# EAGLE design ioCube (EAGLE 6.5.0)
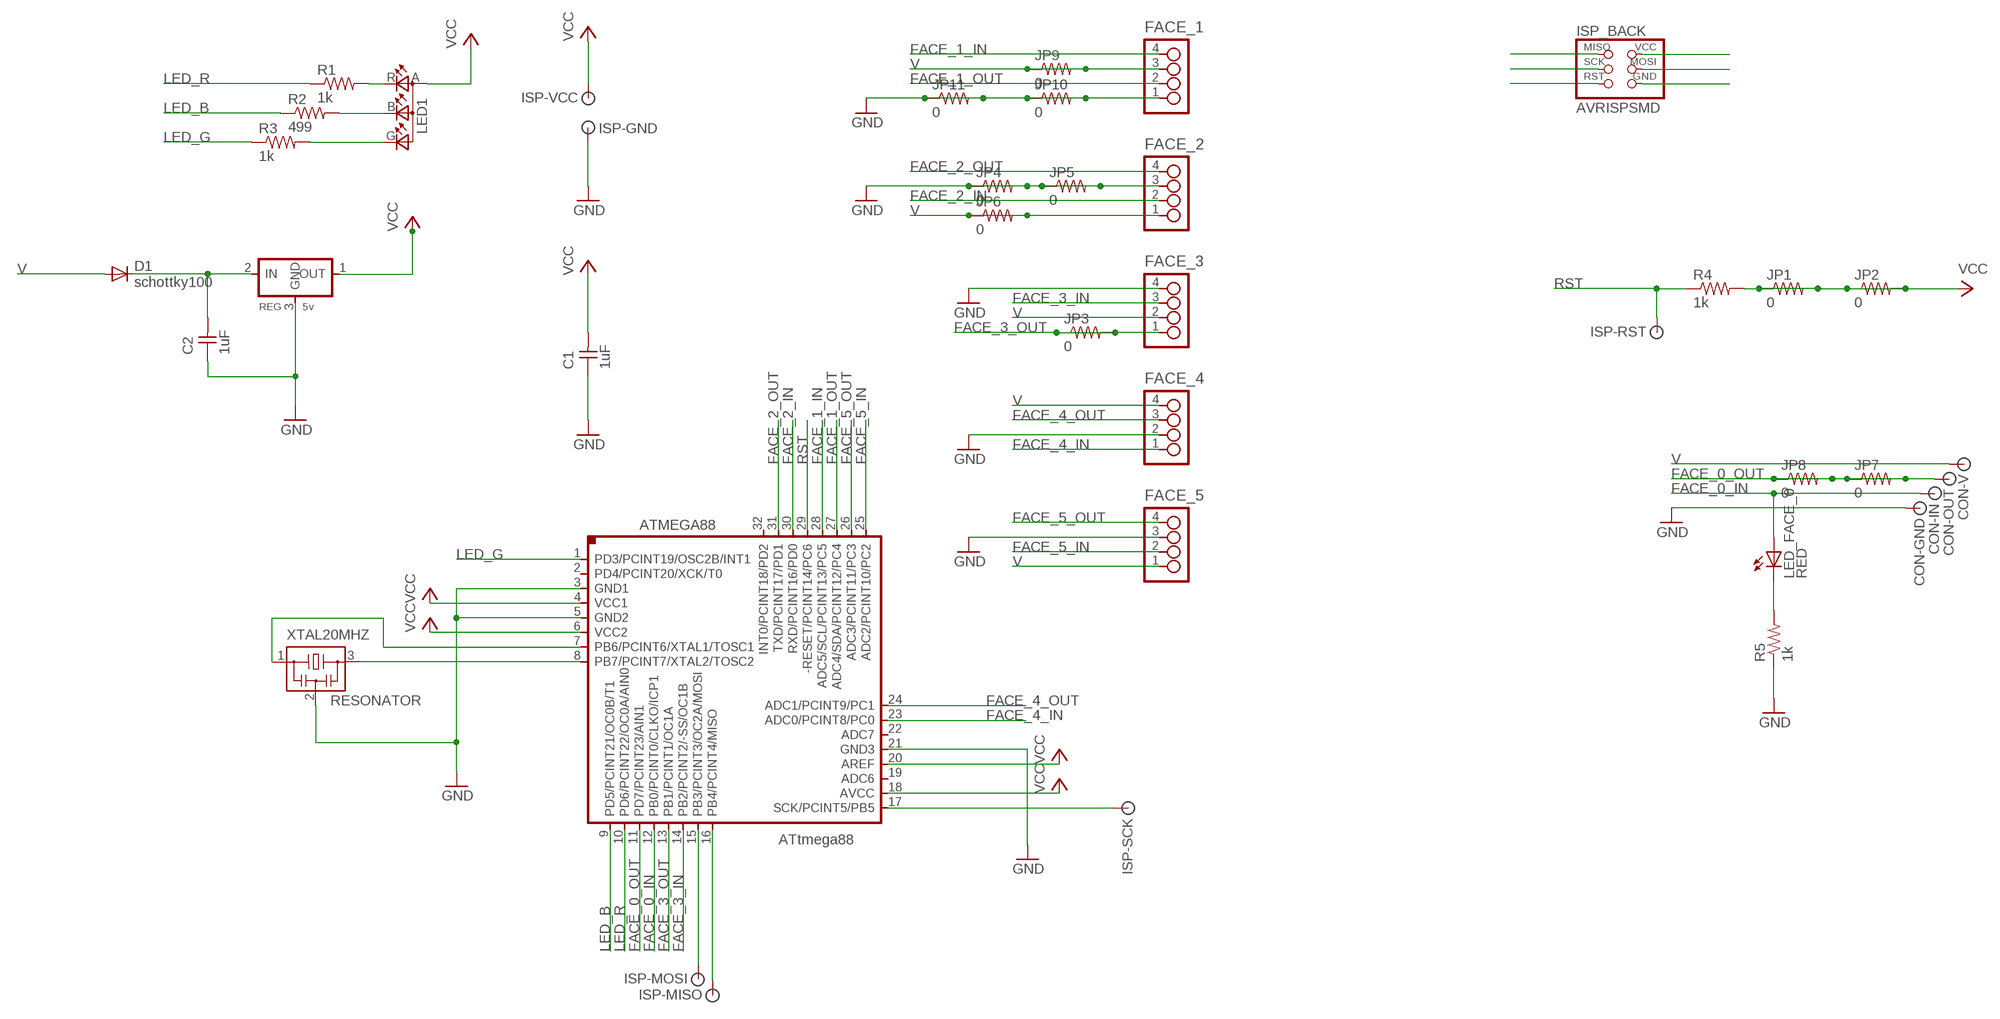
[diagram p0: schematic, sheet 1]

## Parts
ATMEGA88  ATMEGA88TQFP  [TQFP32-08]
C1  1uF  UNPOLARIZED_CAPACITOR1206  [1206]
C2  1uF  UNPOLARIZED_CAPACITOR1206  [1206]
CON-GND  SIGNAL  [PAD.2]
CON-IN  SIGNAL  [PAD.2]
CON-OUT  SIGNAL  [PAD.2]
CON-V  SIGNAL  [PAD.2]
D1  schottky100  DIODESOD123  [SOD123]
FACE_1  4_PIN_HEADER  [SMT_PINS_4]
FACE_2  4_PIN_HEADER  [SMT_PINS_4]
FACE_3  4_PIN_HEADER  [SMT_PINS_4]
FACE_4  4_PIN_HEADER  [SMT_PINS_4]
FACE_5  4_PIN_HEADER  [SMT_PINS_4]
ISP-GND  SIGNAL  [PAD.2]
ISP-MISO  SIGNAL  [PAD.2]
ISP-MOSI  SIGNAL  [PAD.2]
ISP-RST  SIGNAL  [PAD.2]
ISP-SCK  SIGNAL  [PAD.2]
ISP-VCC  SIGNAL  [PAD.2]
ISP_BACK  AVRISPSMD  [2X03SMD]
JP1  0  RESISTOR1206  [1206]
JP2  0  RESISTOR1206  [1206]
JP3  0  RESISTOR1206  [1206]
JP4  0  RESISTOR1206  [1206]
JP5  0  RESISTOR1206  [1206]
JP6  0  RESISTOR1206  [1206]
JP7  0  RESISTOR1206  [1206]
JP8  0  RESISTOR1206  [1206]
JP9  0  RESISTOR1206  [1206]
JP10  0  RESISTOR1206  [1206]
JP11  0  RESISTOR1206  [1206]
LED1  LEDRGBOLD  [P-LCC-4-3]
LED_FACE_0  RED  LED1206  [1206]
R1  1k  RESISTOR1206  [1206]
R2  499  RESISTOR1206  [1206]
R3  1k  RESISTOR1206  [1206]
R4  1k  RESISTOR1206  [1206]
R5  1k  RESISTOR1206  [1206]
REG  5v  REGULATORSOT23  [SOT23]
XTAL20MHZ  RESONATOR  [EFOBM]

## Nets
FACE_0_IN: ATMEGA88.12(PB0/PCINT0/CLKO/ICP1) CON-IN.P$1 LED_FACE_0.1(A)
FACE_0_OUT: ATMEGA88.11(PD7/PCINT23/AIN1) CON-OUT.P$1 JP7.1 JP7.2 JP8.1 JP8.2
FACE_1_IN: ATMEGA88.28(ADC5/SCL/PCINT13/PC5) FACE_1.4
FACE_1_OUT: ATMEGA88.27(ADC4/SDA/PCINT12/PC4) FACE_1.2
FACE_2_IN: ATMEGA88.30(RXD/PCINT16/PD0) FACE_2.2
FACE_2_OUT: ATMEGA88.31(TXD/PCINT17/PD1) FACE_2.4
FACE_3_IN: ATMEGA88.14(PB2/PCINT2/-SS/OC1B) FACE_3.3
FACE_3_OUT: ATMEGA88.13(PB1/PCINT1/OC1A) FACE_3.1 JP3.1 JP3.2
FACE_4_IN: ATMEGA88.23(ADC0/PCINT8/PC0) FACE_4.1
FACE_4_OUT: ATMEGA88.24(ADC1/PCINT9/PC1) FACE_4.3
FACE_5_IN: ATMEGA88.25(ADC2/PCINT10/PC2) FACE_5.2
FACE_5_OUT: ATMEGA88.26(ADC3/PCINT11/PC3) FACE_5.4
GND: ATMEGA88.3(GND1) ATMEGA88.5(GND2) ATMEGA88.21(GND3) C1.1 C2.1 CON-GND.P$1 FACE_1.1 FACE_2.3 FACE_3.4 FACE_4.2 FACE_5.3 ISP-GND.P$1 JP4.1 JP4.2 JP5.1 JP5.2 JP10.1 JP10.2 JP11.1 JP11.2 R5.1 REG.3(GND) XTAL20MHZ.2
LED_B: ATMEGA88.9(PD5/PCINT21/OC0B/T1) R2.1
LED_G: ATMEGA88.1(PD3/PCINT19/OSC2B/INT1) R3.1
LED_R: ATMEGA88.10(PD6/PCINT22/OC0A/AIN0) R1.1
N$1: ATMEGA88.8(PB7/PCINT7/XTAL2/TOSC2) XTAL20MHZ.3
N$2: ATMEGA88.7(PB6/PCINT6/XTAL1/TOSC1) XTAL20MHZ.1
N$3: ATMEGA88.17(SCK/PCINT5/PB5) ISP-SCK.P$1
N$4: ATMEGA88.16(PB4/PCINT4/MISO) ISP-MISO.P$1
N$5: ATMEGA88.15(PB3/PCINT3/OC2A/MOSI) ISP-MOSI.P$1
N$6: LED1.R(CRED) R1.2
N$7: LED_FACE_0.2(C) R5.2
N$8: LED1.B(CBLUE) R2.2
N$9: LED1.G(CGREEN) R3.2
N$10: ISP_BACK.2(VCC)
N$11: C2.2 D1.CATHODE(C) REG.2(IN)
N$12: ISP_BACK.4(MOSI)
N$13: ISP_BACK.6(GND)
N$14: ISP_BACK.1(MISO)
N$15: ISP_BACK.3(SCK)
N$16: ISP_BACK.5(RST)
RST: ATMEGA88.29(-RESET/PCINT14/PC6) ISP-RST.P$1 R4.1
V: CON-V.P$1 D1.ANODE(A) FACE_1.3 FACE_2.1 FACE_3.2 FACE_4.4 FACE_5.1 JP6.1 JP6.2 JP9.1 JP9.2
VCC: ATMEGA88.4(VCC1) ATMEGA88.6(VCC2) ATMEGA88.18(AVCC) ATMEGA88.20(AREF) C1.2 ISP-VCC.P$1 JP1.1 JP1.2 JP2.1 JP2.2 LED1.A(A2) R4.2 REG.1(OUT)
Unconnected: ATMEGA88.2(PD4/PCINT20/XCK/T0) ATMEGA88.19(ADC6) ATMEGA88.22(ADC7) ATMEGA88.32(INT0/PCINT18/PD2)

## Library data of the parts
ATMEGA88 = 01_ng:ATMEGA88
C1 C2 = 01_FAB_Hello:UNPOLARIZED_CAPACITOR: unpolarized_capacitor
CON-GND CON-IN CON-OUT CON-V ISP-GND ISP-MISO ISP-MOSI ISP-RST ISP-SCK ISP-VCC = ot:SIGNAL: Signal
D1 = 01_fab:DIODE: DIODE
FACE_1-FACE_5 = ot:4_PIN_HEADER
ISP_BACK = 01_FAB_Hello:AVRISP
JP1-JP11 R1-R5 = 01_FAB_Hello:RESISTOR
LED1 = fab:LEDRGBOLD: OSRAM Hyper Multi TOPLED® Hyper-Bright LED LATB T686 Source: http://www.osram.convergy.de/
LED_FACE_0 = 01_FAB_Hello:LED
REG = 01_fab:REGULATOR
XTAL20MHZ = 01_fab:RESONATOR

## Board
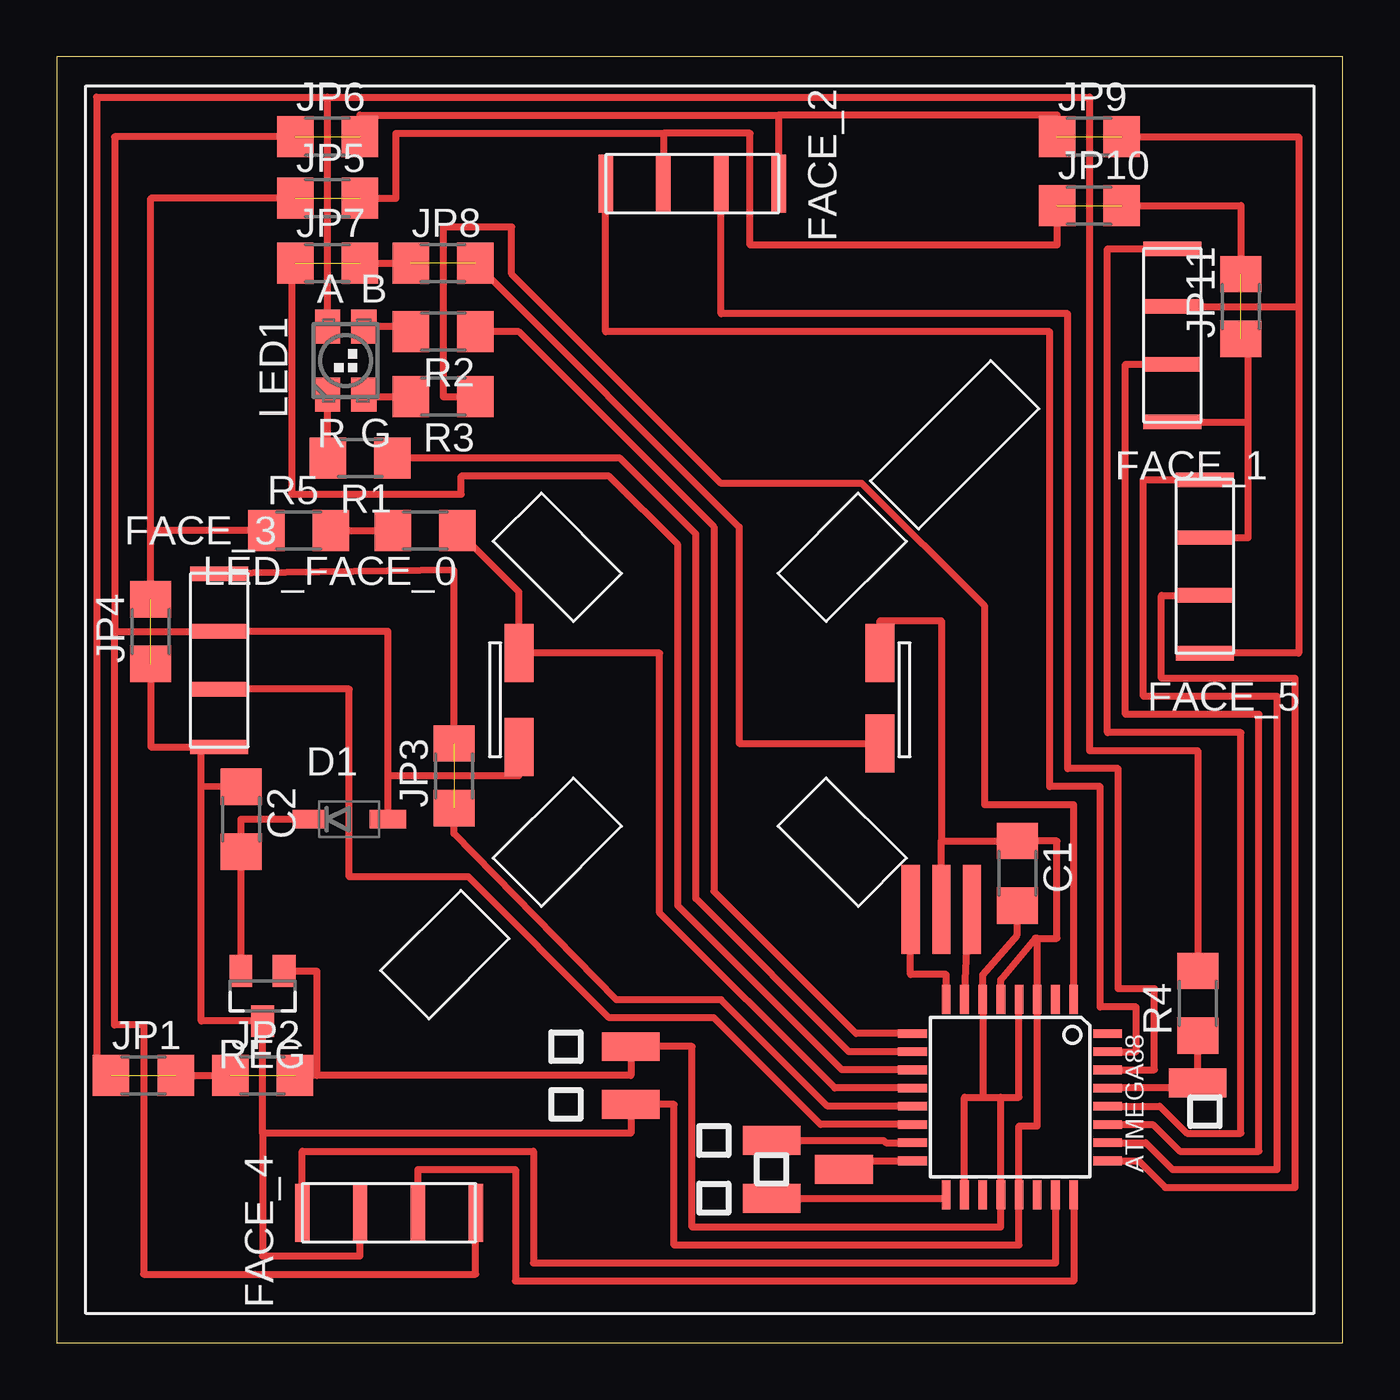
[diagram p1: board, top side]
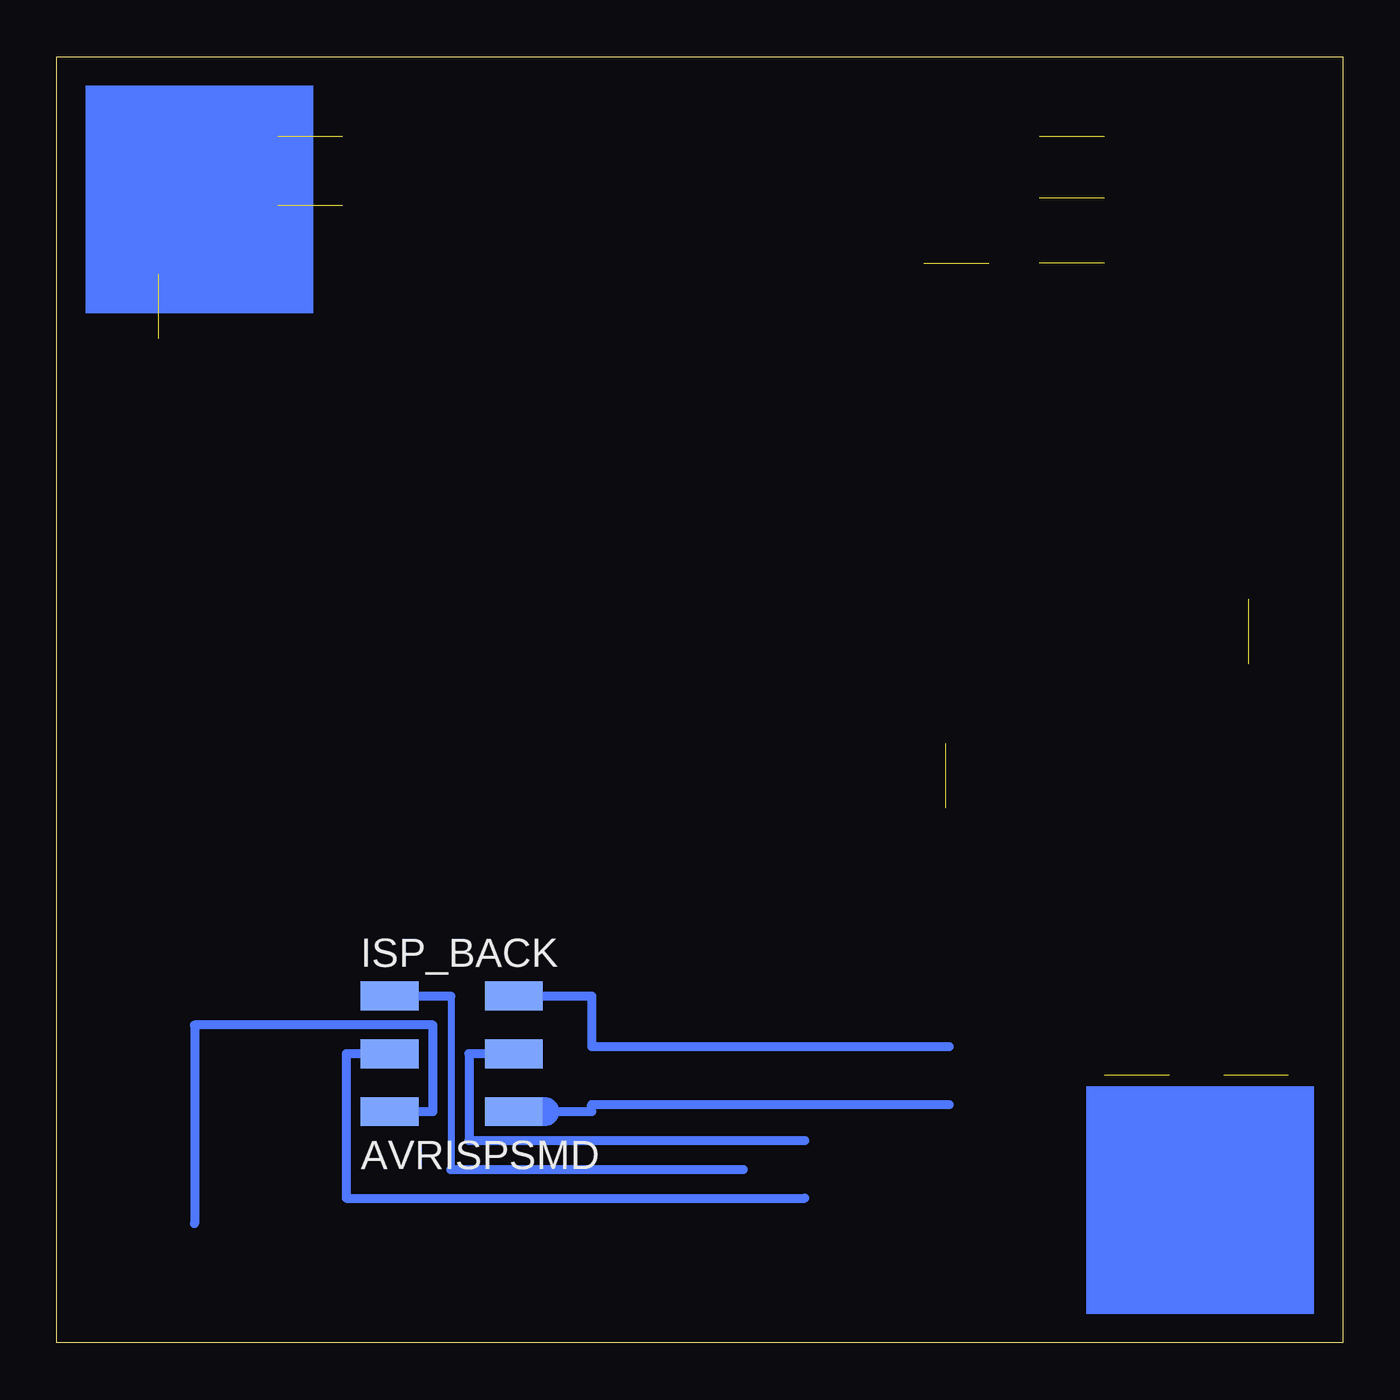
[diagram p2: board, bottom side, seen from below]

Size 56.54 x 56.54 mm. Coordinates in mm from the lower left corner, seen from the top.
Outline: 0,0 56.54,0 56.54,56.54 0,56.54 0,0
Copper layers (1*16): Top 0.035mm / dielectric 1.5mm / Bottom 0.035mm
Design rules "default *": minimum track width 10mil, minimum drill 24mil, track to track 0.4mm, track to pad 0.4mm, pad to pad 0.4mm, via to via 0.4mm, smd to smd 0.4mm, copper to edge 40mil, drill to drill 8mil, minimum pad ring 10mil, minimum via ring 8mil, stop-mask expansion 4mil, vias tented up to drill 0mil, thermal gap 10mil

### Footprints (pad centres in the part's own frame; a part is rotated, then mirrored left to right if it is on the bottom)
TQFP32-08 = smd 1.27 x 0.381: 1 -4.293,2.8; 2 -4.293,2; 3 -4.293,1.2; 4 -4.293,0.4; 5 -4.293,-0.4; 6 -4.293,-1.2; 7 -4.293,-2; 8 -4.293,-2.8; 17 4.293,-2.8; 18 4.293,-2; 19 4.293,-1.2; 20 4.293,-0.4; 21 4.293,0.4; 22 4.293,1.2; 23 4.293,2; 24 4.293,2.8 | smd 0.381 x 1.27: 9 -2.8,-4.293; 10 -2,-4.293; 11 -1.2,-4.293; 12 -0.4,-4.293; 13 0.4,-4.293; 14 1.2,-4.293; 15 2,-4.293; 16 2.8,-4.293; 25 2.8,4.293; 26 2,4.293; 27 1.2,4.293; 28 0.4,4.293; 29 -0.4,4.293; 30 -1.2,4.293; 31 -2,4.293; 32 -2.8,4.293
1206 = smd 1.6 x 1.803: 1 -1.422,0; 2 1.422,0
PAD.2 = smd 2.54 x 1.27: P$1 0,0
SOD123 = smd 1.6 x 0.8: ANODE 1.7,0; CATHODE -1.7,0
SMT_PINS_4 = smd 2.54 x 0.635: 1 0,0; 2 0,2.54; 3 0,5.08; 4 0,7.62
2X03SMD = smd 2.54 x 1.27: 1 -2.54,2.54; 2 2.92,2.54; 3 -2.54,0; 4 2.92,0; 5 -2.54,-2.54; 6 2.92,-2.54
P-LCC-4-3 = smd 1.1 x 1.5: A -0.8,1.5; B 0.8,1.5; G 0.8,-1.5; R -0.8,-1.5
SOT23 = smd 1 x 1.4: 1 -0.95,-1.1; 2 0.95,-1.1; 3 0,1.1
EFOBM = smd 0.8 x 3.9: 1 -1.35,0; 2 0,0; 3 1.35,0

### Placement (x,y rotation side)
ATMEGA88  41.91,10.79 270 top
C1  42.23,20.64 270 top
C2  8.1,23.02 270 top
CON-GND  36.2,30.32 90 top
CON-IN  20.32,30.32 90 top
CON-OUT  36.2,26.35 90 top
CON-V  20.32,26.19 90 top
D1  12.86,23.02 0 top
FACE_1  49.05,40.48 0 top
FACE_2  31.75,50.96 90 top
FACE_3  7.14,33.81 180 top
FACE_4  10.79,5.71 270 top
FACE_5  50.48,30.32 0 top
ISP-GND  25.24,10.48 0 top
ISP-MISO  34.61,7.62 0 top
ISP-MOSI  31.43,8.89 0 top
ISP-RST  50.16,11.43 0 top
ISP-SCK  31.43,6.35 0 top
ISP-VCC  25.24,13.02 0 top
ISP_BACK  39.37,12.7 0 bottom
JP1  3.81,11.75 0 top
JP2  9.05,11.75 0 top
JP3  17.46,24.92 90 top
JP4  4.13,31.27 90 top
JP5  11.91,50.32 0 top
JP6  11.91,53.02 0 top
JP7  11.91,47.47 0 top
JP8  16.99,47.47 0 top
JP9  45.4,53.02 0 top
JP10  45.4,50.01 0 top
JP11  52.07,45.56 90 top
LED1  12.7,43.18 0 top
LED_FACE_0  16.19,35.72 180 top
R1  13.34,38.89 180 top
R2  16.99,44.45 180 top
R3  16.99,41.59 180 top
R4  50.16,14.92 90 top
R5  10.64,35.72 0 top
REG  9.05,15.24 180 top
U$1  [CUBE_NEG]  1.27,1.27 0 top
XTAL20MHZ  38.89,19.05 180 top

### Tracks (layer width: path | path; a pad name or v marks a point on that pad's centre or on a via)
FACE_0_IN
  Top 0.305: ATMEGA88.12 34.21,11.2 26.51,18.89 26.51,30.32 CON-IN.P$1 20.32,33.01 LED_FACE_0.1
FACE_0_OUT  (2 unrouted)
  Top 0.305: ATMEGA88.11 34.52,11.99 27.3,19.21 27.3,35.08 24.29,38.1 17.78,38.1 17.78,37.31 10.32,37.31 10.32,47.47 JP7.1 | JP7.2 JP8.1 | JP8.2 30,35.87 30,26.35 CON-OUT.P$1
FACE_1_IN
  Top 0.305: ATMEGA88.28 48.5,10.39 49.69,9.21 52.07,9.21 52.07,26.83 46.2,26.83 46.2,48.1 FACE_1.4
FACE_1_OUT
  Top 0.305: ATMEGA88.27 48.19,9.6 49.37,8.41 52.86,8.41 52.86,27.62 46.99,27.62 46.99,43.02 FACE_1.2
FACE_2_IN
  Top 0.305: ATMEGA88.30 48.26,11.99 48.26,15.56 46.67,15.56 46.67,25.24 44.45,25.24 44.45,45.24 29.21,45.24 FACE_2.2
FACE_2_OUT
  Top 0.305: ATMEGA88.31 47.47,12.79 47.47,14.76 45.88,14.76 45.88,24.45 43.66,24.45 43.66,44.45 24.13,44.45 FACE_2.4
FACE_3_IN
  Top 0.305: ATMEGA88.14 33.59,9.6 28.89,14.29 24.29,14.29 18.1,20.48 12.86,20.48 12.86,28.73 FACE_3.3
FACE_3_OUT  (1 unrouted)
  Top 0.305: ATMEGA88.13 33.9,10.39 29.21,15.08 24.61,15.08 17.46,22.38 JP3.1 | JP3.2 17.46,33.97 FACE_3.1
FACE_4_IN
  Top 0.305: ATMEGA88.23 43.91,3.49 20.95,3.49 20.95,8.41 10.79,8.41 FACE_4.1
FACE_4_OUT
  Top 0.305: ATMEGA88.24 44.71,2.7 20.16,2.7 20.16,7.62 15.88,7.62 FACE_4.3
FACE_5_IN
  Top 0.305: ATMEGA88.25 47.57,8 48.74,6.83 54.45,6.83 54.45,29.21 48.58,29.21 48.58,32.86 FACE_5.2
FACE_5_OUT
  Top 0.305: ATMEGA88.26 47.88,8.79 49.05,7.62 53.66,7.62 53.66,28.42 47.78,28.42 47.78,37.94 FACE_5.4
GND  (4 unrouted)
  Top 0.305: ATMEGA88.5 41.51,15.95 43.02,17.78 43.11,17.78 | 43.11,17.78 43.97,17.78 43.97,22.06 C1.1 40.79,22.06 38.89,22.07 | 43.11,17.78 ATMEGA88.3 43.11,9.53 42.31,9.53 ATMEGA88.21 42.31,4.29 27.15,4.29 27.15,10.48 ISP-GND.P$1 25.24,9.21 9.05,9.21 | XTAL20MHZ.2 38.89,22.07 | 9.05,9.21 REG.3 6.35,14.14 6.35,24.45 | C2.1 6.35,24.45 | JP4.1 4.13,26.19 FACE_3.4 6.35,26.35 6.35,24.45 | JP4.2 4.13,35.72 | 4.13,35.72 4.13,50.32 JP5.1 | 26.67,53.18 FACE_2.3 | JP5.2 14.92,50.32 14.92,53.18 26.67,53.18 | CON-GND.P$1 36.2,31.75 38.89,31.75 38.89,22.07 | JP10.1 43.98,48.26 30.48,48.26 30.48,53.18 26.67,53.18 | FACE_5.3 52.39,35.4 52.39,40.48 | 52.39,40.48 52.39,44.14 JP11.1 | JP10.2 52.07,50.01 JP11.2 | FACE_1.1 52.39,40.48 | R5.1 4.13,35.72 | 9.05,9.21 9.05,3.81 13.34,3.81 FACE_4.2
LED_B
  Top 0.305: ATMEGA88.9 35.14,13.6 28.89,19.84 28.89,35.88 20.32,44.45 R2.1
LED_G
  Top 0.305: ATMEGA88.1 44.71,23.65 40.8,23.65 40.8,32.38 35.4,37.78 29.21,37.78 20,46.99 20,49.05 16.99,49.05 16.99,41.59 R3.1
LED_R
  Top 0.305: ATMEGA88.10 34.83,12.79 28.1,19.53 28.1,35.56 24.77,38.89 R1.1
N$1
  Top 0.305: ATMEGA88.8 39.11,16.19 37.54,16.19 XTAL20MHZ.3
N$2
  Top 0.305: ATMEGA88.7 40.09,18.58 40.09,18.73 40.01,18.89 XTAL20MHZ.1
N$3
  Top 0.254: 38.95,6.35 ATMEGA88.17
  Top 0.305: ISP-SCK.P$1 38.95,6.35
N$4
  Top 0.305: ISP-MISO.P$1 34.98,8 ATMEGA88.16
N$5
  Top 0.305: ISP-MOSI.P$1 36.35,8.89 36.45,8.79 ATMEGA88.15
N$6
  Top 0.305: R1.2 11.91,41.68 LED1.R
N$7
  Top 0.305: R5.2 LED_FACE_0.2
N$8
  Top 0.305: R2.2 15.56,44.68 LED1.B
N$9
  Top 0.305: LED1.G 13.5,41.59 R3.2
N$11
  Top 0.305: REG.2 8.1,19.05 8.1,20.16 C2.2 8.1,23.02 D1.CATHODE
N$14
  Bottom 0.305: 39.21,15.24 39.21,7.62
  Bottom 0.406: ISP_BACK.1 39.21,15.24 | 39.21,7.62 26.35,7.62
N$15
  Bottom 0.406: ISP_BACK.3 43.81,12.7 43.81,6.35 23.65,6.35
N$16
  Bottom 0.406: ISP_BACK.5 40,10.16 40,13.97 50.48,13.97 50.48,5.24
N$17
  Bottom 0.406: 36.51,12.7 38.42,12.7 38.42,8.89 23.65,8.89
N$18
  Bottom 0.406: 36.35,15.24 33.02,15.24 33.02,13.02 17.3,13.02
N$19
  Bottom 0.305: 36.83,10.16 35.56,10.16
  Bottom 0.406: 35.08,10.16 33.02,10.16 33.02,10.48 17.3,10.48
  Bottom 1.27: 35.56,10.16 35.08,10.16
RST
  Top 0.305: R4.1 ISP-RST.P$1 50.16,11.2 ATMEGA88.29
V  (2 unrouted)
  Top 0.305: 2.54,31.27 2.54,13.97 3.81,13.97 3.81,3.02 18.41,3.02 FACE_4.4 | 2.54,31.27 FACE_3.2 14.56,31.27 14.56,24.92 | D1.ANODE 14.56,24.92 | CON-V.P$1 20.32,24.92 14.56,24.92 | FACE_2.1 31.75,53.98 | JP6.1 2.54,53.02 2.54,31.27 | JP6.2 13.33,53.98 31.75,53.98 | JP9.1 43.98,53.98 31.75,53.98 | JP9.2 54.61,53.02 54.61,45.56 | 54.61,45.56 54.61,30.32 FACE_5.1 | FACE_1.3 54.61,45.56
VCC  (2 unrouted)
  Top 0.305: ATMEGA88.18 39.91,10.79 40.71,10.79 | 40.71,10.79 41.51,10.79 | 41.51,10.79 42.31,10.79 ATMEGA88.4 | 41.51,10.79 ATMEGA88.20 41.51,5.08 27.94,5.08 27.94,13.02 ISP-VCC.P$1 25.24,11.75 11.43,11.75 | 40.71,10.79 ATMEGA88.6 40.71,16.19 42.23,17.94 C1.2 | 11.43,11.75 JP2.2 | REG.1 11.43,16.34 11.43,11.75 | JP1.2 JP2.1 | 11.9,54.77 1.75,54.77 1.75,11.75 JP1.1 | 11.9,54.77 45.4,54.77 45.4,26.04 50.16,26.04 R4.2 | LED1.A 11.9,54.77
(copper drawn outside any net)
  shapes: Bottom area x2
